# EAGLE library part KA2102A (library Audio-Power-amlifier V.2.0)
http://www.datasheetcatalog.org/datasheet/SamsungElectronic/mXuztvq.pdf
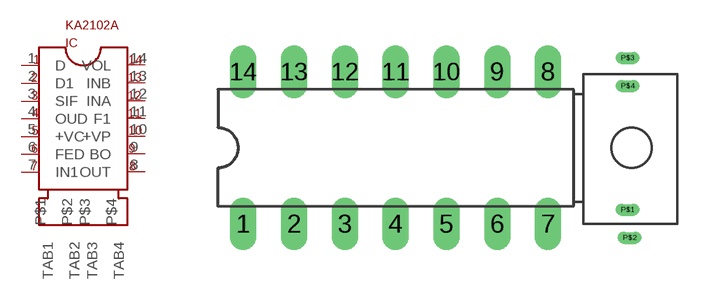
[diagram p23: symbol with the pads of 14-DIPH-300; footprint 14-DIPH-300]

Designator prefix IC

## KA2102A  [14-DIPH-300]
1  D
2  D1
3  SIF
4  OUD  out
5  +VC  pwr
6  FED
7  IN1
8  OUT  out
9  BO
10  +VP  pwr
11  F1
12  INA
13  INB
14  VOL
P$1  TAB1
P$2  TAB2
P$3  TAB3
P$4  TAB4

## Footprint 14-DIPH-300 (pad centres in mm)
Dual In Line Package
drill 0.813 long: 1 -7.62,-3.81; 2 -5.08,-3.81; 3 -2.54,-3.81; 4 0,-3.81; 5 2.54,-3.81; 6 5.08,-3.81; 7 7.62,-3.81; 8 7.62,3.81; 9 5.08,3.81; 10 2.54,3.81; 11 0,3.81; 12 -2.54,3.81; 13 -5.08,3.81; 14 -7.62,3.81
drill 0 pad 0.61 long: P$1 11.6,-3.1; P$2 11.7,-4.5; P$3 11.6,4.5; P$4 11.6,3.1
